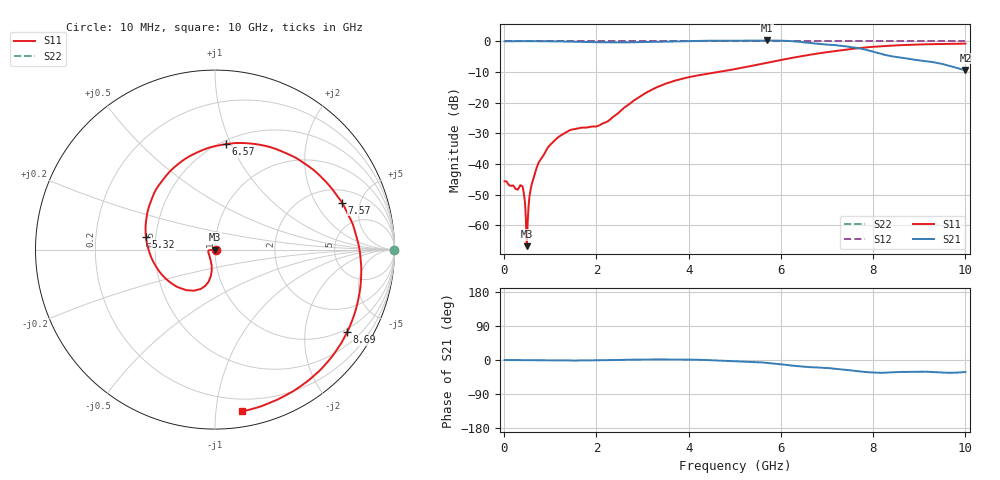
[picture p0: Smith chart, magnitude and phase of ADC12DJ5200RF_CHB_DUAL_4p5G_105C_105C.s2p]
! Texas Instruments, Inc.
! ADC12DJ5200RF - CH B S-Parameters (Dual Ch Mode, Fs = 4.5 GSPS, 105 degC case, 105 degC juntion)
! Port 1 represents the 100-ohm differenal input, Port 2 the digital output
! freq  dbS11  angS11  dbS21 angS21 dbS12 angS12 dbS22 angS22
# HZ S DB R 100
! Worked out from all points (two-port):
!   1000 points, 10 MHz to 10 GHz, reference 100 ohm
!   highest |S21| = 0.25 dB at 5.69 GHz (marker M1); lowest = -9.4 dB at 10 GHz (marker M2)
!   |S21| within 3 dB of the highest: start of sweep to 7.831 GHz
!   lowest |S11| = -66.8 dB at 490 MHz (marker M3), VSWR 1.00, Z = 100 + j0.0909 ohm
!   |S11| at or under -10 dB: start of sweep to 4.655 GHz
!   |S22| runs from 0.0 to 0.0 dB; largest |S21 - S12| = 0.73
!   S11 on the Smith chart (normalised r, x): 10 MHz: 1.01, -0.00; 5.32 GHz: 0.44, +0.07; 6.57 GHz: 0.53, +0.96; 7.57 GHz: 2.79, +3.39; 8.69 GHz: 0.87, -3.26; 10 GHz: 0.11, -1.18
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1e7  -45.69 -2.8  0.00 -0.0  0.00 0.0  0.00 0.0
3.8e8  -47.17 -16.4  0.02 -0.3  0.00 0.0  0.00 0.0
4.9e8  -66.84 93.5  0.02 -0.4  0.00 0.0  0.00 0.0
5.2e8  -56.15 -177.4  0.02 -0.4  0.00 0.0  0.00 0.0
5.8e8  -47.93 -158.5  0.03 -0.5  0.00 0.0  0.00 0.0
6.5e8  -44.16 -162.0  0.01 -0.6  0.00 0.0  0.00 0.0
9.2e8  -35.36 -172.3  0.02 -0.9  0.00 0.0  0.00 0.0
1.25e9  -30.53 -174.5  -0.08 -1.5  0.00 0.0  0.00 0.0
1.68e9  -28.19 -167.0  -0.24 -1.3  0.00 0.0  0.00 0.0
2.22e9  -26.31 -127.8  -0.34 -0.7  0.00 0.0  0.00 0.0
3.34e9  -14.84 -101.2  -0.18 1.4  0.00 0.0  0.00 0.0
4.23e9  -11.08 -126.9  0.09 0.6  0.00 0.0  0.00 0.0
5.01e9  -9.07 -169.7  0.18 -3.2  0.00 0.0  0.00 0.0
5.32e9  -8.17 169.9  0.16 -4.5  0.00 0.0  0.00 0.0
5.69e9  -7.06 144.7  0.25 -7.6  0.00 0.0  0.00 0.0
6.57e9  -4.57 84.1  -0.45 -18.2  0.00 0.0  0.00 0.0
6.67e9  -4.31 77.3  -0.63 -19.1  0.00 0.0  0.00 0.0
7.09e9  -3.36 49.3  -1.15 -22.0  0.00 0.0  0.00 0.0
7.57e9  -2.45 20.4  -1.98 -28.1  0.00 0.0  0.00 0.0
8.34e9  -1.48 -18.1  -4.72 -32.9  0.00 0.0  0.00 0.0
8.69e9  -1.23 -32.1  -5.55 -31.6  0.00 0.0  0.00 0.0
1e10  -0.78 -80.5  -9.40 -31.6  0.00 0.0  0.00 0.0
